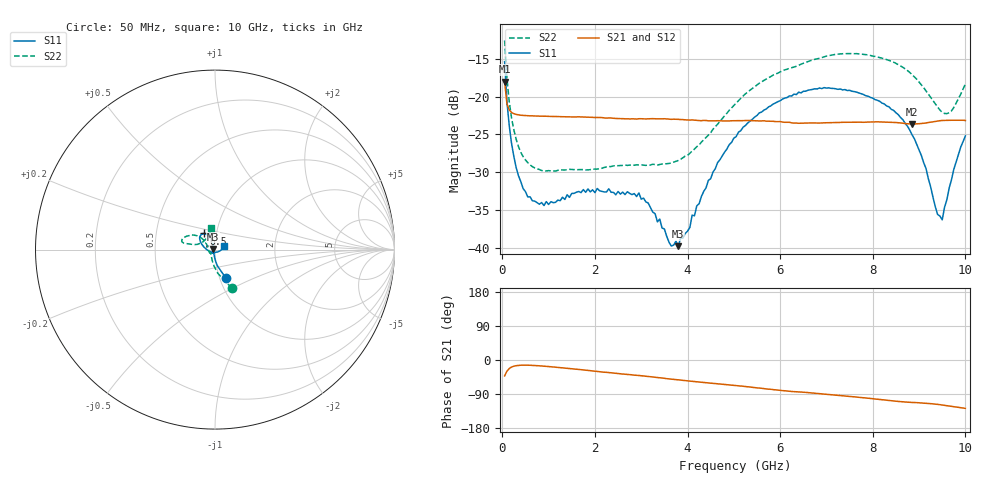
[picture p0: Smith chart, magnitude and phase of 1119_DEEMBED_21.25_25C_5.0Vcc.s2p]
!Hittite Microwave Corp.
!Digital Attenuator/PhaseShifter Rev 1.4.0
!Filename: C:\DATA\DATA\1119_DEEMBED_21.25_25C_5.0Vcc.s2p
!VNA ID: Agilent Technologies,N5224A,MY51441122,A.10.45.03
!Device type:
!2 Port Calibration.
!Temp(C): 25
!Lot Number:
!Serial Number:
!Operator:
!Misc:
!Attenuator:  21.250
# GHZ S DB R 50.0
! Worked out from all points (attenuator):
!   200 points, 50 MHz to 10 GHz, reference 50 ohm
!   highest |S21| = -18.02 dB at 50 MHz (marker M1); lowest = -23.6 dB at 8.85 GHz (marker M2)
!   lowest |S11| = -39.8 dB at 3.8 GHz (marker M3), VSWR 1.02, Z = 49 + j0.283 ohm
!   |S11| at or under -10 dB: start of sweep to end of sweep
!   |S22| runs from -29.8 to -12.6 dB; largest |S21 - S12| = 0.00024
!   S11 on the Smith chart (normalised r, x): 50 MHz: 1.07, -0.35; 6.5 GHz: 0.87, +0.16; 10 GHz: 1.11, +0.04
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0.05  -15.40 -69.2  -18.02 -42.0  -18.02 -42.0  -12.60 -66.5
0.1  -20.65 -81.3  -20.95 -29.6  -20.95 -29.6  -17.55 -83.4
0.2  -26.19 -91.1  -22.11 -18.6  -22.11 -18.6  -22.84 -100.1
0.35  -30.46 -98.8  -22.42 -14.2  -22.43 -14.2  -26.62 -114.1
0.55  -33.24 -107.5  -22.53 -13.7  -22.52 -13.7  -28.72 -125.7
0.9  -34.39 -115.4  -22.60 -16.2  -22.60 -16.2  -29.81 -134.9
1.75  -32.28 -125.6  -22.70 -26.2  -22.71 -26.2  -29.65 -139.6
2.95  -32.73 -123.9  -22.93 -40.9  -22.94 -41.0  -29.03 -158.6
3.4  -36.17 -143.8  -22.94 -46.8  -22.95 -46.9  -28.97 -172.0
3.65  -39.73 -171.0  -23.01 -50.3  -23.02 -50.4  -28.77 179.0
3.8  -39.75 163.7  -23.01 -52.5  -23.02 -52.5  -28.44 172.2
4.65  -28.71 107.2  -23.19 -62.7  -23.21 -62.7  -23.65 143.1
5.05  -25.29 108.4  -23.19 -67.4  -23.21 -67.4  -20.84 139.6
5.55  -22.16 113.1  -23.23 -74.1  -23.24 -74.1  -18.25 141.9
6.5  -19.31 124.0  -23.52 -84.9  -23.53 -84.9  -15.61 152.1
6.7  -19.06 127.2  -23.48 -87.1  -23.49 -87.1  -15.17 154.5
8.35  -21.36 155.0  -23.40 -106.8  -23.40 -106.7  -15.23 168.0
8.85  -25.07 171.0  -23.63 -112.0  -23.63 -112.0  -17.12 167.7
9.400001  -35.56 -110.0  -23.24 -117.0  -23.25 -117.0  -21.39 153.5
9.5  -36.27 -67.9  -23.16 -118.8  -23.18 -118.8  -22.10 144.1
9.7  -30.98 -15.4  -23.13 -122.2  -23.15 -122.2  -21.89 121.0
10  -25.19 21.1  -23.16 -127.7  -23.16 -127.7  -18.35 99.5
